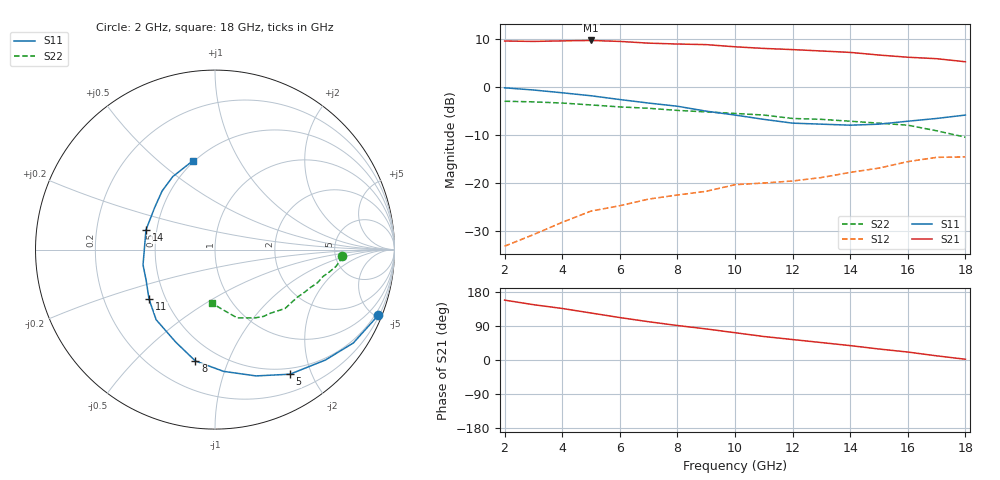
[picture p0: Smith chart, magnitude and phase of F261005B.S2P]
!ATF-26100
!S-PARAMETERS at Vds=5V  Id=30mA.  LAST UPDATED 07-22-92
# ghz s ma r 50
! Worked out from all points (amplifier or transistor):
!   17 points, 2 GHz to 18 GHz, reference 50 ohm
!   highest |S21| = 9.7 dB at 5 GHz (marker M1)
!   |S21| within 3 dB of that: start of sweep to 14.93 GHz
!   unconditionally stable (mu >= 1): 8.09 GHz to 15.89 GHz; 17.7 GHz to end of sweep
!   at 4 GHz: K = 0.64, MSG = 18.9 dB, |S12| = -28.2 dB
!   at 10 GHz: K = 1.05, MAG = 13.0 dB, |S12| = -20.4 dB
!   at 18 GHz: K = 1.02, MAG = 9.1 dB, |S12| = -14.6 dB
!   S11 on the Smith chart (normalised r, x): 2 GHz: 0.28, -5.13; 5 GHz: 0.42, -1.69; 8 GHz: 0.37, -0.77; 11 GHz: 0.41, -0.28; 14 GHz: 0.44, +0.11; 18 GHz: 0.49, +0.66
2  0.98 -22.0  3.01 158.0  0.022 85.0  0.71 -3.0
3  0.93 -34.0  2.98 146.0  0.029 81.0  0.7 -5.0
4  0.87 -45.0  3.02 136.0  0.039 78.0  0.68 -8.0
5  0.81 -59.0  3.05 124.0  0.051 76.0  0.65 -11.0
6  0.74 -72.0  2.98 112.0  0.058 74.0  0.62 -14.0
7  0.68 -86.0  2.86 101.0  0.068 72.0  0.6 -18.0
8  0.63 -100.0  2.8 91.0  0.075 70.0  0.57 -22.0
9  0.56 -113.0  2.76 82.0  0.082 69.0  0.55 -26.0
10  0.51 -130.0  2.62 72.0  0.096 68.0  0.53 -30.0
11  0.46 -143.0  2.52 62.0  0.1 66.0  0.51 -40.0
12  0.42 -156.0  2.45 54.0  0.105 64.0  0.47 -49.0
13  0.41 -168.0  2.37 46.0  0.114 60.0  0.46 -54.0
14  0.4 164.0  2.29 38.0  0.129 56.0  0.44 -60.0
15  0.41 145.0  2.15 29.0  0.143 52.0  0.42 -65.0
16  0.44 132.0  2.04 21.0  0.167 45.0  0.4 -72.0
17  0.47 120.0  1.97 11.0  0.185 40.0  0.35 -80.0
18  0.51 104.0  1.83 2.0  0.187 34.0  0.3 -93.0
